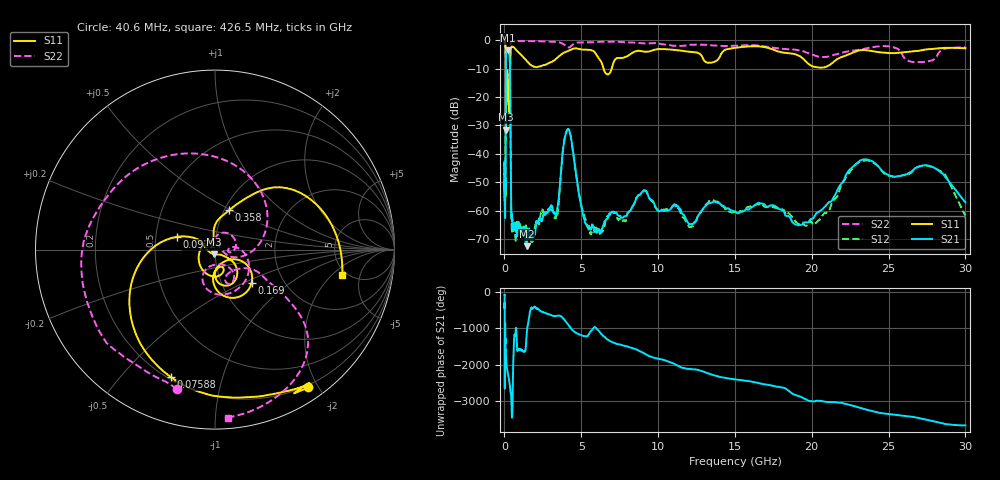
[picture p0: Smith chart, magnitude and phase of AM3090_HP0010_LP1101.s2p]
! Date/Time: Thu, Feb 28, 2019 1:55 PM
! Network Analyzer: Agilent Technologies E8364B Rev: A.07.50.67
! Sweep from 0.010 to 30.000 GHz, 1601 Points, Sweep Type: LOG
! Power Supply: 5.023 V, 0.002 A
# Hz S DB R 50
!freq MagS11 AngS11 MagS21 AngS21 MagS12 AngS12 MagS22 AngS22
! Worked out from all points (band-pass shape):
!   1601 points, 10 MHz to 30 GHz, reference 50 ohm
!   highest |S21| = -3.56 dB at 235.1 MHz (marker M1); lowest = -72.5 dB at 1.446 GHz (marker M2)
!   |S21| within 3 dB of the highest: 102.5 MHz to 343.9 MHz (241.4 MHz wide, 108 % of centre)
!   lowest |S11| = -31.5 dB at 99.92 MHz (marker M3), VSWR 1.05, Z = 49.4 - j2.55 ohm
!   |S11| at or under -10 dB: 90.68 MHz to 369.7 MHz (279 MHz wide, 121 % of centre); 6.45 GHz to 6.98 GHz (529.5 MHz wide, 7.89 % of centre)
!   |S22| runs from -32.6 to -0.1 dB; largest |S21 - S12| = 0.012
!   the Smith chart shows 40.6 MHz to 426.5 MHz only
!   S11 on the Smith chart (normalised r, x): 40.6 MHz: 0.17, -1.88; 75.88 MHz: 0.21, -0.69; 92.24 MHz: 0.65, +0.10; 169 MHz: 1.38, -0.55; 358 MHz: 1.05, +0.49; 426.5 MHz: 4.59, -2.68
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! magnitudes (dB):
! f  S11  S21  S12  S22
! 10 MHz  -0.3  -45.3  -43.2  -0.7
! 38.04 MHz  -0.5  -59.3  -61.7  -1.7
! 40.6 MHz  -0.7  -60.8  -61.0  -1.9
! 75.88 MHz  -2.5  -46.4  -45.8  -4.4
! 92.24 MHz  -13.0  -13.9  -14.0  -13.4
! 99.92 MHz  -31.5  -7.4  -7.4  -32.2
! 115 MHz  -13.8  -4.9  -4.9  -19.1
! 144.7 MHz  -20.0  -3.7  -3.6  -22.2
! 169 MHz  -11.2  -3.6  -3.6  -13.6
! 235.1 MHz  -20.0  -3.6  -3.5  -17.8
! 358 MHz  -12.7  -8.7  -8.7  -8.5
! 426.5 MHz  -2.8  -53.5  -52.6  -0.6
! 550.5 MHz  -2.4  -65.6  -65.3  -0.2
! 1.446 GHz  -7.3  -72.5  -66.5  -0.3
! 2.084 GHz  -9.5  -64.1  -63.8  -0.4
! 3.385 GHz  -6.4  -61.5  -62.7  -0.7
! 4.115 GHz  -3.9  -31.4  -31.3  -2.5
! 5.528 GHz  -3.4  -65.7  -67.8  -0.8
! 7.926 GHz  -5.8  -61.9  -63.2  -0.8
! 19.7 GHz  -7.9  -64.2  -65.2  -4.5
! 23.48 GHz  -3.5  -42.0  -42.4  -3.0
! 30 GHz  -2.9  -57.0  -61.7  -2.5
